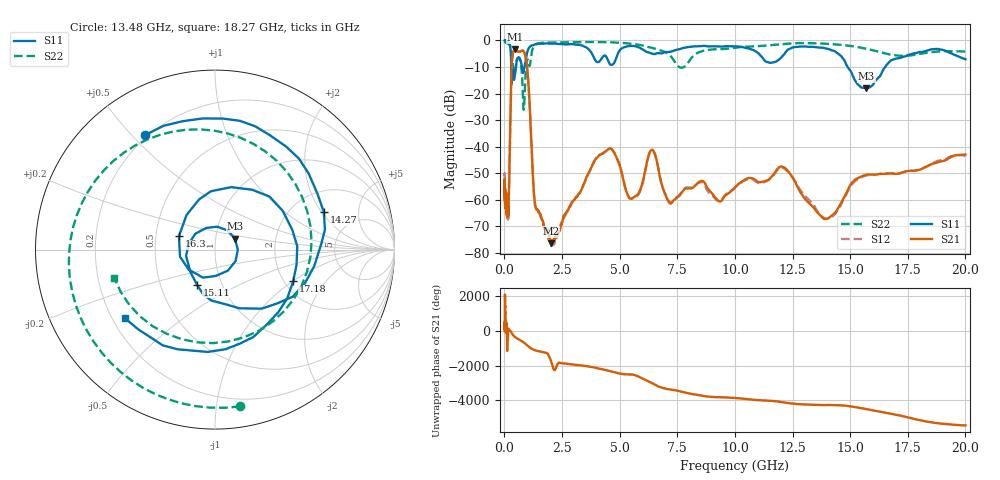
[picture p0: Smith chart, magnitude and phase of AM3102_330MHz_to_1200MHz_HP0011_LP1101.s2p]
! Date/Time: Tue, Sep 11, 2018 5:12 PM
! Network Analyzer: Agilent Technologies E8362B Rev: A.07.50.63
! Sweep from 0.010 to 20.000 GHz, 1601 Points, Sweep Type: LOG
! Power Supply: 4.949 V, 0.001 A
# Hz S DB R 50
!freq MagS11 AngS11 MagS21 AngS21 MagS12 AngS12 MagS22 AngS22
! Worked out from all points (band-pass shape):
!   1601 points, 10 MHz to 20 GHz, reference 50 ohm
!   highest |S21| = -3.29 dB at 464.5 MHz (marker M1); lowest = -76.4 dB at 2.016 GHz (marker M2)
!   |S21| within 3 dB of the highest: 342.3 MHz to 924 MHz (581.7 MHz wide, 91.9 % of centre)
!   lowest |S11| = -18.0 dB at 15.7 GHz (marker M3), VSWR 1.29, Z = 62 + j7.59 ohm
!   |S11| at or under -10 dB: 298.8 MHz to 500.8 MHz (202 MHz wide, 50.5 % of centre); 758.7 MHz to 870.2 MHz (111.4 MHz wide, 13.7 % of centre); 14.89 GHz to 16.52 GHz (1.624 GHz wide, 10.3 % of centre)
!   |S22| runs from -26.1 to -0.3 dB; largest |S21 - S12| = 0.012
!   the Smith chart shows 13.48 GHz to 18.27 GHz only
!   S11 on the Smith chart (normalised r, x): 13.48 GHz: 0.19, +0.55; 14.27 GHz: 2.96, +2.10; 15.11 GHz: 0.76, -0.31; 16.3 GHz: 0.66, +0.10; 17.18 GHz: 2.23, -1.01; 18.27 GHz: 0.25, -0.32
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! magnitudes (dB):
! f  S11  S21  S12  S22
! 10 MHz  0.0  -53.2  -52.0  -0.3
! 35.55 MHz  0.0  -58.2  -61.8  -0.6
! 126.4 MHz  -0.4  -61.3  -62.8  -1.1
! 175.4 MHz  -0.9  -65.2  -62.9  -1.3
! 313.2 MHz  -15.5  -9.9  -9.9  -5.0
! 447.2 MHz  -13.6  -3.3  -3.4  -12.2
! 464.5 MHz  -12.7  -3.3  -3.3  -11.5
! 942.8 MHz  -6.6  -7.2  -7.3  -10.3
! 1.302 GHz  -1.6  -59.6  -60.4  -1.9
! 1.59 GHz  -1.3  -66.2  -66.5  -0.9
! 2.016 GHz  -1.2  -76.4  -76.5  -0.8
! 4.479 GHz  -7.2  -41.2  -41.1  -0.6
! 5.652 GHz  -2.1  -58.8  -59.1  -1.4
! 6.396 GHz  -5.0  -41.2  -41.6  -2.8
! 13.48 GHz  -2.5  -63.7  -63.0  -1.1
! 14.27 GHz  -3.9  -65.6  -66.0  -1.4
! 15.11 GHz  -13.2  -53.3  -53.9  -2.2
! 15.7 GHz  -18.0  -50.6  -50.9  -3.1
! 16.3 GHz  -13.4  -50.3  -50.2  -4.4
! 17.18 GHz  -6.6  -50.1  -49.9  -5.8
! 18.27 GHz  -4.0  -47.7  -47.7  -4.7
! 20 GHz  -7.1  -43.0  -43.5  -4.2
